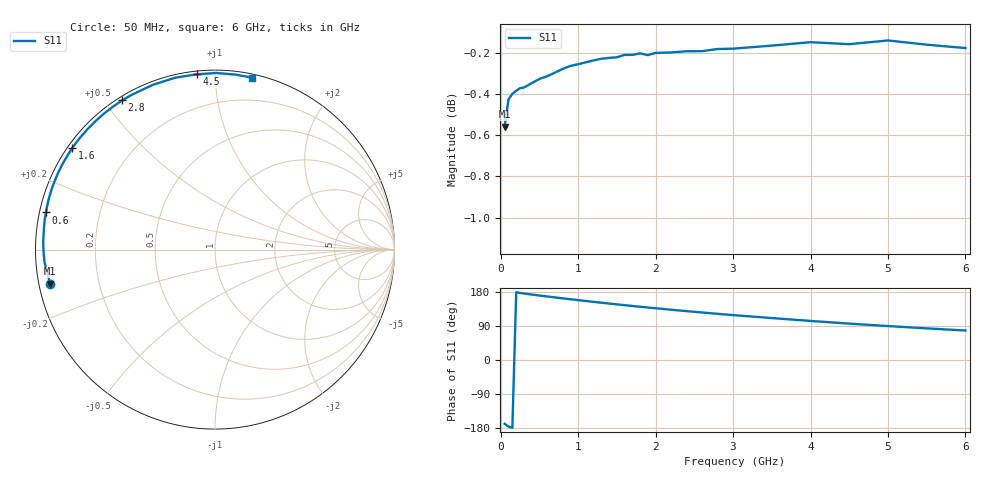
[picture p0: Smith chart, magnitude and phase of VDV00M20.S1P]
! Infineon Technologies  Discrete & RF Semiconductors
! BBY 55-03
! Si Tuning Diode in SOD323
! VR =
! S-Parameters:  June  1999
# GHz  S  MA  R  50
!  f  S11
! GHz  MAG  ANG
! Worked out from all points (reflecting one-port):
!   34 points, 50 MHz to 6 GHz, reference 50 ohm
!   lowest |S11| = -0.6 dB at 50 MHz (marker M1), VSWR 31.12, Z = 1.62 - j5.12 ohm
!   phase of S11 starts at -168 deg and turns -114 deg over the sweep
!   S11 on the Smith chart (normalised r, x): 50 MHz: 0.03, -0.10; 600 MHz: 0.02, +0.11; 1.6 GHz: 0.01, +0.32; 2.8 GHz: 0.01, +0.56; 4.5 GHz: 0.02, +0.90; 6 GHz: 0.03, +1.24
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0.05  0.9377 -168.3
0.1  0.9522 -175.7
0.15  0.9551 -178.9
0.2  0.9568 178.9
0.25  0.9582 177.1
0.3  0.9585 175.5
0.4  0.9609 172.7
0.6  0.9646 167.6
0.8  0.9686 162.7
0.9  0.9702 160.4
1  0.9711 158.0
1.2  0.9732 153.4
1.4  0.9745 149.0
1.6  0.9762 144.7
1.7  0.9762 142.5
1.8  0.977 140.5
2  0.9773 136.6
2.2  0.9775 132.7
2.4  0.9782 129.0
2.6  0.9782 125.4
2.8  0.9794 121.9
3  0.9796 118.5
3.5  0.9813 110.7
4  0.9831 103.1
4.5  0.982 96.0
5  0.9841 89.6
5.5  0.9818 83.4
6  0.9799 77.9
